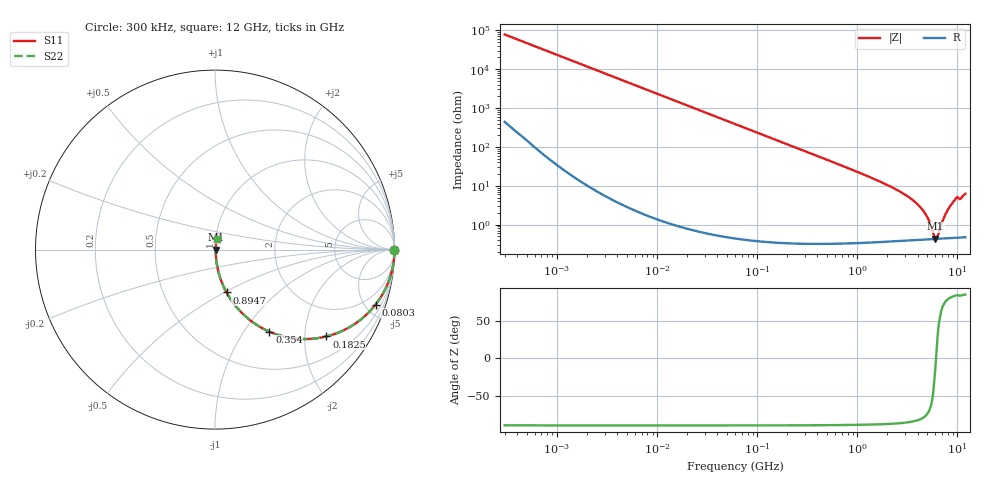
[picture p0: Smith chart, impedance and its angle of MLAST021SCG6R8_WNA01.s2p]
! MLAST021SCG6R8_WNA01  S-PARAMETER MODEL  ( General Type )
! Model Generated by TAIYO YUDEN Corporation (http://www.ty-top.com)
! Version 1.0
! TAIYO YUDEN Control No. 220901
! Copyright(c) 2022 TAIYO YUDEN CO.,LTD. All Rights Reserved.
! Product Description (link to TY-COMPAS)
! https://ds.yuden.co.jp/TYCOMPAS/or/detail?pn=MLAST021SCG6R8CWNA01&u=M
! Products Name : Multilayer Ceramic Capacitors
! Characteristics :
!  Capacitance : 6.8 pF , Rated Voltage : 25V , TCC : CG / C0G
!  Case Size : 0.25 x 0.125 / 0.0098 x 0.0049 [mm/inch] , Thickness : 0.125 / 0.0049 [mm/inch]
!  (Conditions: Temperature = 25 degC , DC Bias Current/Voltage = 0A / 0V)
! External Node Assignments :
!  1  o---| |---o  2
! GND o---------o GND
! Frequency Range : 0.3MHz  -  12000MHz  [ 401 STEP ]
# MHz S RI R 50
! Freq[MHz].  S11 Real  S11 Imag  S21 Real  S21 Imag  S12 Real  S12 Imag  S22 Real  S22 Imag
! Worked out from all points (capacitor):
!   401 points, 300 kHz to 12 GHz, reference 50 ohm
!   read as one part in series: C = 6.8 pF near 316.3 kHz
!   lowest |Z| = 439 mohm at 6.026 GHz (marker M1)
!   series resonance near 6.106 GHz, so ESL is about 100 pH
!   S11 on the Smith chart (normalised r, x): 300 kHz: open; 80.3 MHz: 1.01, -5.83; 182.5 MHz: 1.01, -2.56; 354 MHz: 1.01, -1.32; 894.7 MHz: 1.01, -0.51; 12 GHz: 1.01, +0.12
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0.3  1 -0.00128  8.89e-06 0.00128  8.89e-06 0.00128  1 -0.00128
1.769972  0.9999 -0.00756  6.42e-05 0.00756  6.42e-05 0.00756  0.9999 -0.00756
10.44266  0.998 -0.0445  0.00201 0.0445  0.00201 0.0445  0.998 -0.0445
27.10171  0.9867 -0.1142  0.0133 0.1142  0.0133 0.1142  0.9867 -0.1142
60  0.9381 -0.2404  0.0619 0.2404  0.0619 0.2404  0.9381 -0.2404
80.29859  0.8943 -0.3067  0.1057 0.3067  0.1057 0.3067  0.8943 -0.3067
119.4772  0.7927 -0.4044  0.2073 0.4044  0.2073 0.4044  0.7927 -0.4044
182.544  0.621 -0.4838  0.379 0.4838  0.379 0.4838  0.621 -0.4838
353.9943  0.3036 -0.4574  0.6964 0.4574  0.6964 0.4574  0.3036 -0.4574
555.3718  0.1506 -0.3538  0.8494 0.3538  0.8494 0.3538  0.1506 -0.3538
894.6982  0.0642 -0.2387  0.9358 0.2387  0.9358 0.2387  0.0642 -0.2387
2088.533  0.0132 -0.0971  0.9868 0.0971  0.9868 0.0971  0.0132 -0.0971
3107.553  0.00692 -0.0549  0.9931 0.0549  0.9931 0.0549  0.00692 -0.0549
4158.869  0.00494 -0.0295  0.9951 0.0295  0.9951 0.0295  0.00494 -0.0295
5006.236  0.00439 -0.0148  0.9956 0.0148  0.9956 0.0148  0.00439 -0.0148
5715.274  0.00428 -0.00453  0.9957 0.00453  0.9957 0.00453  0.00428 -0.00453
6026.253  0.00429 -0.000842  0.9957 0.000842  0.9957 0.000842  0.00429 -0.000842
6354.153  0.00433 0.00271  0.9957 -0.00271  0.9957 -0.00271  0.00433 0.00271
7448.838  0.00468 0.016  0.9953 -0.016  0.9953 -0.016  0.00468 0.016
8732.115  0.00563 0.0332  0.9944 -0.0332  0.9944 -0.0332  0.00563 0.0332
9708.23  0.00687 0.0475  0.9931 -0.0475  0.9931 -0.0475  0.00687 0.0475
12000  0.00851 0.0613  0.9915 -0.0613  0.9915 -0.0613  0.00851 0.0613
